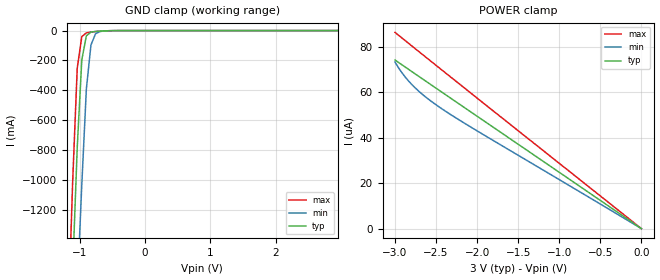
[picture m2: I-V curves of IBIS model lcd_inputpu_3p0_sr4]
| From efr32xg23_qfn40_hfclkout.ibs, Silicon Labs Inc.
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|   Model lcd_inputpu_3p0_sr4
[Model]  lcd_inputpu_3p0_sr4
Model_type Input
C_comp   1.6300pF   1.4000pF   2.7000pF
[Temperature Range]   25.0000   0.1250k   -40.0000
[Pullup Reference]   3.0000V   2.7000V   3.3000V
[Pulldown Reference]   0.0V   0.0V   0.0V
[POWER Clamp Reference]   3.0000V   2.7000V   3.3000V
[GND Clamp Reference]   0.0V   0.0V   0.0V
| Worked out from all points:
|   GND clamp passes 1 mA (typ) near -0.55 V on its own axis
[GND_clamp]
|Voltage   I(typ)   I(min)   I(max)
-3V       -24.27A    -21.95A    -26.57A
-1.18V    -2.447A    -3.183A    -1.952A
-1.11V    -1.614A    -2.464A    -1.015A
-1.04V    -784.1mA   -1.746A    -252.9mA
-970mV    -196.3mA   -1.031A    -40.14mA
-900mV    -35.08mA   -390.8mA   -15.06mA
-830mV    -10.42mA   -97.01mA   -10.06mA
-760mV    -5.797mA   -21.5mA    -6.671mA
-690mV    -3.556mA   -6.118mA   -3.988mA
-340mV    -93.05uA   -110.6uA   -107.9uA
2.95V     -1.243uA   5.421uA    -10.07uA
[POWER_clamp]
|Voltage   I(typ)   I(min)   I(max)
-3V       74.15uA    73.25uA    86.28uA
-2.88V    71.16uA    66.87uA    82.79uA
-2.76V    68.19uA    62.1uA     79.31uA
-2.6V     64.23uA    57.12uA    74.68uA
-2.44V    60.27uA    52.96uA    70.06uA
-2V       49.42uA    42.99uA    57.39uA
0V        741.4pA    8.424nA    1.116nA
